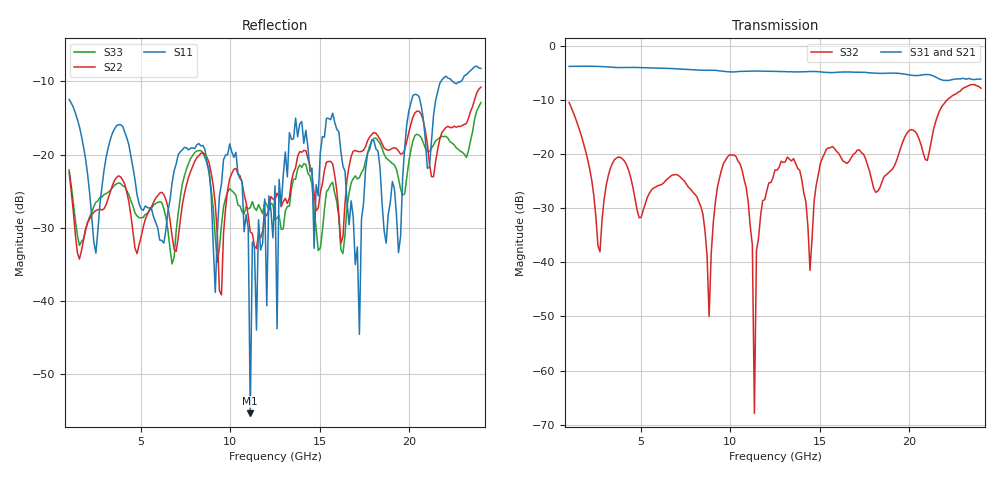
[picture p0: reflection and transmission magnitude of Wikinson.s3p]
! MDIF file - written using SXPWrite.m
# GHz S RI R 50
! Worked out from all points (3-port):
!   201 points, 1 GHz to 24 GHz, reference 50 ohm
!   strongest paths, dB at 1 GHz, 6.75 GHz, 12.5 GHz, 18.25 GHz, 24 GHz:
!     S31: -3.8, -4.2, -4.7, -5.1, -6.2
!     S21: -3.8, -4.3, -4.8, -5.2, -6.3
!     S32: -10.5, -23.9, -22.9, -26.8, -7.9
!   lowest |S11| = -55.3 dB at 11.12 GHz (marker M1), VSWR 1.00, Z = 50 - j0.167 ohm
!   |S11| at or under -10 dB: start of sweep to 21.78 GHz; 22.41 GHz to 22.89 GHz (478.4 MHz wide, 2.11 % of centre)
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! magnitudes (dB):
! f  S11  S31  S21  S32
! 1 GHz  -12.5  -3.8  -3.8  -10.5
! 8.82 GHz  -22.2  -4.5  -4.6  -50.0
! 10.31 GHz  -19.7  -4.8  -4.8  -20.4
! 11.12 GHz  -55.3  -4.7  -4.7  -33.4
! 11.35 GHz  -32.6  -4.7  -4.7  -67.9
! 11.46 GHz  -44.0  -4.7  -4.7  -37.8
! 12.5 GHz  -24.3  -4.7  -4.8  -22.9
! 15.72 GHz  -14.4  -5.0  -5.0  -18.6
! 17.21 GHz  -44.5  -4.9  -5.0  -19.2
! 24 GHz  -8.3  -6.2  -6.3  -7.9
